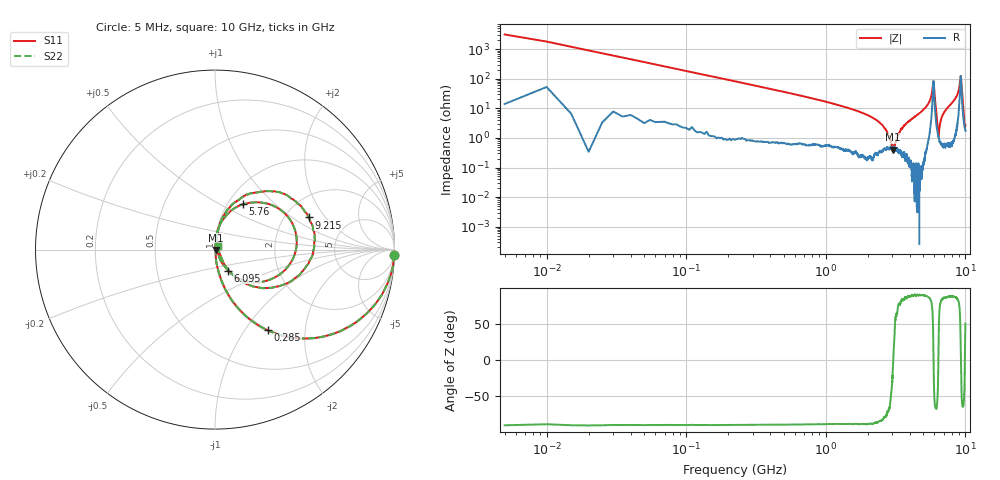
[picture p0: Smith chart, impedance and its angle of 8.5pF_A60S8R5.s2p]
! Amotech Co.,Ltd.
! http://www.amotech.co.kr/
! Part Number: A60S8R5
! These Parameters are Measured in Series Mode Connection
! Operation Temp=25[degC], DC Bias Voltage=0[V]
! Freq. Start=5[MHz] Stop=10[GHz], 2000[Steps]
! Date: Monday, July 13, 2020, 01:33:34
# GHZ S RI R 50.000000
!Freq.(Hz) S11(Real) S11(Imag) S21(Real) S21(Imag) S12(Real) S12(Imag) S22(Real) S22(Imag)
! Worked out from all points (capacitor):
!   2000 points, 5 MHz to 10 GHz, reference 50 ohm
!   read as one part in series: C = 8.68 pF near 55 MHz
!   lowest |Z| = 404 mohm at 3.005 GHz (marker M1)
!   series resonance near 3.038 GHz, so ESL is about 320 pH
!   S11 on the Smith chart (normalised r, x): 5 MHz: 1, -63; 285 MHz: 1.02, -1.28; 5.76 GHz: 1.17, +0.65; 6.095 GHz: 1.12, -0.27; 9.215 GHz: 2.67, +1.37; 10 GHz: 1.03, +0.04
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0.005  0.9988 -0.0318  0.00116 0.0318  0.00116 0.0318  0.9988 -0.0318
0.1  0.767 -0.4168  0.233 0.4168  0.233 0.4168  0.767 -0.4168
0.285  0.2943 -0.4492  0.7057 0.4492  0.7057 0.4492  0.2943 -0.4492
0.66  0.0728 -0.2481  0.9272 0.2481  0.9272 0.2481  0.0728 -0.2481
1.675  0.00979 -0.0811  0.9902 0.0811  0.9902 0.0811  0.00979 -0.0811
2.54  0.00452 -0.027  0.9955 0.027  0.9955 0.027  0.00452 -0.027
3.005  0.00364 -0.00172  0.9964 0.00172  0.9964 0.00172  0.00364 -0.00172
3.34  0.00351 0.0138  0.9965 -0.0138  0.9965 -0.0138  0.00351 0.0138
3.81  0.00312 0.032  0.9969 -0.032  0.9969 -0.032  0.00312 0.032
5.005  0.00928 0.0895  0.9907 -0.0895  0.9907 -0.0895  0.00928 0.0895
5.76  0.1553 0.2519  0.8447 -0.2519  0.8447 -0.2519  0.1553 0.2519
5.915  0.4485 -0.0113  0.5515 0.0113  0.5515 0.0113  0.4485 -0.0113
6.095  0.0722 -0.1166  0.9278 0.1166  0.9278 0.1166  0.0722 -0.1166
6.4  0.0109 -0.00101  0.9891 0.00101  0.9891 0.00101  0.0109 -0.00101
6.67  0.00829 0.0387  0.9917 -0.0387  0.9917 -0.0387  0.00829 0.0387
7.1  0.0115 0.077  0.9885 -0.077  0.9885 -0.077  0.0115 0.077
8.335  0.0436 0.1821  0.9564 -0.1821  0.9564 -0.1821  0.0436 0.1821
8.915  0.1596 0.2971  0.8404 -0.2971  0.8404 -0.2971  0.1596 0.2971
9.215  0.522 0.1791  0.478 -0.1791  0.478 -0.1791  0.522 0.1791
9.41  0.2958 -0.2138  0.7042 0.2138  0.7042 0.2138  0.2958 -0.2138
9.89  0.023 -0.00869  0.977 0.00869  0.977 0.00869  0.023 -0.00869
10  0.0171 0.0198  0.9829 -0.0198  0.9829 -0.0198  0.0171 0.0198
